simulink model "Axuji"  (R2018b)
settings: Solver=VariableStepAuto  StartTime=0.0  StopTime=1  RelTol=1e-3
libraries: fuzblock x6

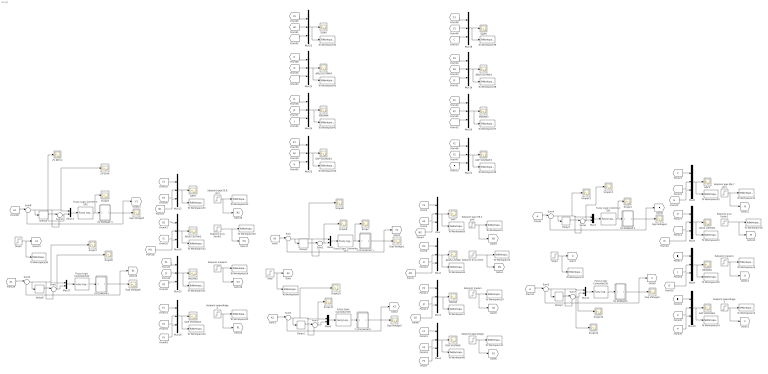
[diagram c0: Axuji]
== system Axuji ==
  2V EDMGAP 3 : Subsystem
  2V EDMGAP3 : Subsystem
  2V Error : Scope
  2V dError : Scope
  3.5V EDMGAP 1 : Subsystem
  3.5V EDMGAP2 : Subsystem
  5V EDMGAP 2 : Subsystem
  5V EDMGAP1 : Subsystem
  ARUS LISTRIK{,1..4} (5 alike) : Scope
  Delay{1..6} (6 alike) : Delay  DelayLength=1
  From11 : From
  From8 : From
  Fuzzy Logic Controller 3X1 : fuzblock/Fuzzy Logic  Controller  FIS=FixFUZZYSUGENO3X3  OutputSampleNumber=101  DataType=double  FuzzifiedInputs=off  RuleFiringStrengths=off  RuleOutputs=off  AggregatedOutputs=off  SimulateUsing=Interpreted execution  OutOfRangeInputValueMessage=warning  NoRuleFiredMessage=warning  EmptyOutputFuzzySetMessage=warning
  Fuzzy Logic Controller 3X2 : fuzblock/Fuzzy Logic  Controller  FIS=FixFUZZYSUGENO3X3  OutputSampleNumber=101  DataType=double  FuzzifiedInputs=off  RuleFiringStrengths=off  RuleOutputs=off  AggregatedOutputs=off  SimulateUsing=Interpreted execution  OutOfRangeInputValueMessage=warning  NoRuleFiredMessage=warning  EmptyOutputFuzzySetMessage=warning
  Fuzzy Logic Controller 3X3 : fuzblock/Fuzzy Logic  Controller  FIS=FixFUZZYSUGENO3X3  OutputSampleNumber=101  DataType=double  FuzzifiedInputs=off  RuleFiringStrengths=off  RuleOutputs=off  AggregatedOutputs=off  SimulateUsing=Interpreted execution  OutOfRangeInputValueMessage=warning  NoRuleFiredMessage=warning  EmptyOutputFuzzySetMessage=warning
  Fuzzy Logic Controller5X1 : fuzblock/Fuzzy Logic  Controller  FIS=FixFUZZYSUGENO5X5  OutputSampleNumber=101  DataType=double  FuzzifiedInputs=off  RuleFiringStrengths=off  RuleOutputs=off  AggregatedOutputs=off  SimulateUsing=Interpreted execution  OutOfRangeInputValueMessage=warning  NoRuleFiredMessage=warning  EmptyOutputFuzzySetMessage=warning
  Fuzzy Logic Controller5X2 : fuzblock/Fuzzy Logic  Controller  FIS=FixFUZZYSUGENO5X5  OutputSampleNumber=101  DataType=double  FuzzifiedInputs=off  RuleFiringStrengths=off  RuleOutputs=off  AggregatedOutputs=off  SimulateUsing=Interpreted execution  OutOfRangeInputValueMessage=warning  NoRuleFiredMessage=warning  EmptyOutputFuzzySetMessage=warning
  Fuzzy Logic Controller5X5 : fuzblock/Fuzzy Logic  Controller  FIS=FixFUZZYSUGENO5X5  OutputSampleNumber=101  DataType=double  FuzzifiedInputs=off  RuleFiringStrengths=off  RuleOutputs=off  AggregatedOutputs=off  SimulateUsing=Interpreted execution  OutOfRangeInputValueMessage=warning  NoRuleFiredMessage=warning  EmptyOutputFuzzySetMessage=warning
  GAP{,1..4} (5 alike) : Scope
  GAP VOLTAGE{,1..4} (5 alike) : Scope
  Gap Voltage{1..6} (6 alike) : Scope
  Goto7 : Goto
  MEDAN{,1..4} (5 alike) : Scope
  Mux{,2..4,6,8..10,12,14..16,18..25} (20 alike) : Mux  Inputs=3
  Mux{1,5,7,11,13,17} (6 alike) : Mux  Inputs=2
  Scope{,1..2,6..15} (13 alike) : Scope
  Setpoint arus listrik : Step  Time=0  After=0.00246  SampleTime=0
  Setpoint arus listrik1 : Step  Time=0  After=0.00246  SampleTime=0
  Setpoint arus listrik2 : Step  Time=0  After=0.00246  SampleTime=0
  Setpoint gap (59,3 µm) : Step  Time=0  After=59.3  SampleTime=0
  Setpoint gap (84,7 µm) : Step  Time=0  After=84.7  SampleTime=0
  Setpoint gap(33,8 µm) : Step  Time=0  After=33.8  SampleTime=0
  Setpoint gapvoltage : Step  Time=0  After=2  SampleTime=0
  Setpoint gapvoltage1 : Step  Time=0  After=2  SampleTime=0
  Setpoint gapvoltage2 : Step  Time=0  After=2  SampleTime=0
  Setpoint medan : Step  Time=0  After=59000  SampleTime=0
  Setpoint medan1 : Step  Time=0  After=59000  SampleTime=0
  Setpoint medan2 : Step  Time=0  After=59000  SampleTime=0
  Step : Step  Time=0  After=3.5  SampleTime=0
  Step1 : Step  Time=0  After=5  SampleTime=0
  Step2 : Step  Time=0  After=2  SampleTime=0
  Sum{,1..11} (12 alike) : Sum  Inputs=|-+
  To Workspace1 : ToWorkspace  VariableName=setpointgap  SaveFormat=Timeseries  SampleTime=-1
  To Workspace10 : ToWorkspace  VariableName=setpointmedan  SaveFormat=Timeseries  SampleTime=-1
  To Workspace11 : ToWorkspace  VariableName=setpointgvoltage  SaveFormat=Timeseries  SampleTime=-1
  To Workspace12 : ToWorkspace  VariableName=setpointgap1  SaveFormat=Timeseries  SampleTime=-1
  To Workspace13 : ToWorkspace  VariableName=setpointmedan1  SaveFormat=Timeseries  SampleTime=-1
  To Workspace14 : ToWorkspace  VariableName=setpointgvoltage1  SaveFormat=Timeseries  SampleTime=-1
  To Workspace17 : ToWorkspace  VariableName=setpoint1  SaveFormat=Timeseries  SampleTime=-1
  To Workspace18 : ToWorkspace  VariableName=setpointaruslistrik1  SaveFormat=Timeseries  SampleTime=-1
  To Workspace19 : ToWorkspace  VariableName=gapvoltage10  SaveFormat=Timeseries  SampleTime=-1
  To Workspace20 : ToWorkspace  VariableName=medan10  SaveFormat=Timeseries  SampleTime=-1
  To Workspace21 : ToWorkspace  VariableName=aruslistrik10  SaveFormat=Timeseries  SampleTime=-1
  To Workspace22 : ToWorkspace  VariableName=gap10  SaveFormat=Timeseries  SampleTime=-1
  To Workspace23 : ToWorkspace  VariableName=setpointgap2  SaveFormat=Timeseries  SampleTime=-1
  To Workspace24 : ToWorkspace  VariableName=setpointmedan2  SaveFormat=Timeseries  SampleTime=-1
  To Workspace25 : ToWorkspace  VariableName=setpointgvoltage2  SaveFormat=Timeseries  SampleTime=-1
  To Workspace28 : ToWorkspace  VariableName=setpoint2  SaveFormat=Timeseries  SampleTime=-1
  To Workspace29 : ToWorkspace  VariableName=setpointaruslistrik2  SaveFormat=Timeseries  SampleTime=-1
  To Workspace30 : ToWorkspace  VariableName=gapvoltage8  SaveFormat=Timeseries  SampleTime=-1
  To Workspace31 : ToWorkspace  VariableName=medan8  SaveFormat=Timeseries  SampleTime=-1
  To Workspace32 : ToWorkspace  VariableName=aruslistrik8  SaveFormat=Timeseries  SampleTime=-1
  To Workspace33 : ToWorkspace  VariableName=gap8  SaveFormat=Timeseries  SampleTime=-1
  To Workspace36 : ToWorkspace  VariableName=gapvoltage6  SaveFormat=Timeseries  SampleTime=-1
  To Workspace37 : ToWorkspace  VariableName=medan6  SaveFormat=Timeseries  SampleTime=-1
  To Workspace38 : ToWorkspace  VariableName=aruslistrik6  SaveFormat=Timeseries  SampleTime=-1
  To Workspace39 : ToWorkspace  VariableName=gap6  SaveFormat=Timeseries  SampleTime=-1
  To Workspace4 : ToWorkspace  VariableName=setpoint  SaveFormat=Timeseries  SampleTime=-1
  To Workspace40 : ToWorkspace  VariableName=gapvoltage7  SaveFormat=Timeseries  SampleTime=-1
  To Workspace41 : ToWorkspace  VariableName=medan7  SaveFormat=Timeseries  SampleTime=-1
  To Workspace42 : ToWorkspace  VariableName=aruslistrik7  SaveFormat=Timeseries  SampleTime=-1
  To Workspace43 : ToWorkspace  VariableName=gap7  SaveFormat=Timeseries  SampleTime=-1
  To Workspace5 : ToWorkspace  VariableName=setpointaruslistrik  SaveFormat=Timeseries  SampleTime=-1
  To Workspace6 : ToWorkspace  VariableName=gapvoltage9  SaveFormat=Timeseries  SampleTime=-1
  To Workspace7 : ToWorkspace  VariableName=medan9  SaveFormat=Timeseries  SampleTime=-1
  To Workspace8 : ToWorkspace  VariableName=aruslistrik9  SaveFormat=Timeseries  SampleTime=-1
  To Workspace9 : ToWorkspace  VariableName=gap9  SaveFormat=Timeseries  SampleTime=-1
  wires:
  [N2] -> Mux/3
  Setpoint gapvoltage/1 -> [P2], To Workspace11/1
  [I2] -> Mux2/2
  [D2] -> Mux2/1
  Sum2/1 -> Scope9/1, Mux1/2
  Mux5/1 -> Fuzzy Logic Controller5X5/1
  [O2] -> Mux3/3
  Delay2/1 -> Sum3/1
  [H2] -> Mux/2
  Mux/1 -> To Workspace9/1, GAP/1
  Setpoint arus listrik/1 -> [M2], To Workspace5/1
  Setpoint medan/1 -> [O2], To Workspace10/1
  Sum/1 -> Delay1/1, Scope8/1, Sum2/2, Mux1/1
  [M2] -> Mux2/3
  Delay1/1 -> Sum2/1
  [K2] -> Mux4/2
  [J2] -> Mux3/2
  [F2] -> Mux4/1
  Mux1/1 -> Fuzzy Logic Controller 3X3/1
  Fuzzy Logic Controller 3X3/1 -> Scope/1, 3.5V EDMGAP 1/1(In1)
  Mux4/1 -> To Workspace6/1, GAP VOLTAGE/1
  [A2] -> Sum1/1
  Setpoint gap (59,3 µm)/1 -> [N2], To Workspace1/1
  Mux3/1 -> To Workspace7/1, MEDAN/1
  [E2] -> Mux3/1
  Sum1/1 -> Delay2/1, Scope10/1, Sum3/2, Mux5/1
  Step/1 -> To Workspace4/1, [A2]
  Mux2/1 -> To Workspace8/1, ARUS LISTRIK/1
  Sum3/1 -> Scope11/1, Mux5/2
  [C2] -> Mux/1
  [A2] -> Sum/1
  [P2] -> Mux4/3
  3.5V EDMGAP2/1(Out1) -> [K2], Gap Voltage2/1, Sum1/2
  3.5V EDMGAP 1/1(Out1) -> Sum/2, Gap Voltage1/1, [F2]
  Fuzzy Logic Controller5X5/1 -> 3.5V EDMGAP2/1(In1)
  5V EDMGAP1/1(Out1) -> [K], Gap Voltage4/1, Sum5/2
  [J] -> Mux9/2
  Setpoint gapvoltage1/1 -> [P], To Workspace14/1
  Fuzzy Logic Controller5X1/1 -> 5V EDMGAP1/1(In1)
  [H] -> Mux6/2
  [N] -> Mux6/3
  [C] -> Mux6/1
  Mux6/1 -> To Workspace22/1, GAP1/1
  [F] -> Mux10/1
  Sum7/1 -> Scope15/1, Mux11/2
  Mux9/1 -> To Workspace20/1, MEDAN1/1
  Mux8/1 -> To Workspace21/1, ARUS LISTRIK1/1
  Sum5/1 -> Delay4/1, Sum7/2, Scope14/1, Mux11/1
  [P] -> Mux10/3
  Mux7/1 -> Fuzzy Logic Controller 3X1/1
  [O] -> Mux9/3
  Step1/1 -> To Workspace17/1, Goto7/1
  From11/1 -> Sum5/1
  [I] -> Mux8/2
  Mux10/1 -> To Workspace19/1, GAP VOLTAGE1/1
  Fuzzy Logic Controller 3X1/1 -> Scope1/1, 5V EDMGAP 2/1(In1)
  [K] -> Mux10/2
  [M] -> Mux8/3
  Setpoint arus listrik1/1 -> [M], To Workspace18/1
  Delay3/1 -> Sum6/1
  Setpoint gap (84,7 µm)/1 -> [N], To Workspace12/1
  5V EDMGAP 2/1(Out1) -> Sum4/2, Gap Voltage3/1, [F]
  [E] -> Mux9/1
  Delay4/1 -> Sum7/1
  Sum6/1 -> Scope13/1, Mux7/2
  Setpoint medan1/1 -> [O], To Workspace13/1
  From8/1 -> Sum4/1
  [D] -> Mux8/1
  Sum4/1 -> Delay3/1, Scope12/1, Sum6/2, Mux7/1
  Mux11/1 -> Fuzzy Logic Controller5X1/1
  2V EDMGAP3/1(Out1) -> [K1], Gap Voltage6/1, Sum9/2
  [J1] -> Mux15/2
  Setpoint gapvoltage2/1 -> [P1], To Workspace25/1
  Fuzzy Logic Controller5X2/1 -> 2V EDMGAP3/1(In1)
  [H1] -> Mux12/2
  [N1] -> Mux12/3
  [C1] -> Mux12/1
  Mux12/1 -> To Workspace33/1, GAP2/1
  [F1] -> Mux16/1
  Sum11/1 -> Scope6/1, Mux17/2
  Mux15/1 -> To Workspace31/1, MEDAN2/1
  Mux14/1 -> To Workspace32/1, ARUS LISTRIK2/1
  Sum9/1 -> Delay6/1, Sum11/2, Scope7/1, Mux17/1
  [P1] -> Mux16/3
  Mux13/1 -> Fuzzy Logic Controller 3X2/1
  [O1] -> Mux15/3
  Step2/1 -> To Workspace28/1, [A1]
  [A1] -> Sum9/1
  [I1] -> Mux14/2
  Mux16/1 -> To Workspace30/1, GAP VOLTAGE2/1
  Fuzzy Logic Controller 3X2/1 -> Scope2/1, 2V EDMGAP 3/1(In1)
  [K1] -> Mux16/2
  [M1] -> Mux14/3
  Setpoint arus listrik2/1 -> [M1], To Workspace29/1
  Delay5/1 -> Sum10/1
  Setpoint gap(33,8 µm)/1 -> [N1], To Workspace23/1
  2V EDMGAP 3/1(Out1) -> Sum8/2, Gap Voltage5/1, [F1]
  [E1] -> Mux15/1
  Delay6/1 -> Sum11/1
  Sum10/1 -> 2V dError/1, Mux13/2
  Setpoint medan2/1 -> [O1], To Workspace24/1
  [A1] -> Sum8/1
  [D1] -> Mux14/1
  Sum8/1 -> Delay5/1, Sum10/2, 2V Error/1, Mux13/1
  Mux17/1 -> Fuzzy Logic Controller5X2/1
  [D2] -> Mux19/2
  [F1] -> Mux21/1
  Mux21/1 -> To Workspace36/1, GAP VOLTAGE3/1
  Mux20/1 -> To Workspace37/1, MEDAN3/1
  Mux18/1 -> To Workspace39/1, GAP3/1
  [F] -> Mux21/3
  [C2] -> Mux18/2
  [E2] -> Mux20/2
  [F2] -> Mux21/2
  [E1] -> Mux20/1
  [D] -> Mux19/3
  [C] -> Mux18/3
  Mux19/1 -> To Workspace38/1, ARUS LISTRIK3/1
  [E] -> Mux20/3
  [C1] -> Mux18/1
  [D1] -> Mux19/1
  [I2] -> Mux23/2
  [K1] -> Mux25/1
  Mux25/1 -> To Workspace40/1, GAP VOLTAGE4/1
  Mux24/1 -> To Workspace41/1, MEDAN4/1
  Mux22/1 -> To Workspace43/1, GAP4/1
  [K] -> Mux25/3
  [H2] -> Mux22/2
  [J2] -> Mux24/2
  [K2] -> Mux25/2
  [J1] -> Mux24/1
  [I] -> Mux23/3
  [H] -> Mux22/3
  Mux23/1 -> To Workspace42/1, ARUS LISTRIK4/1
  [J] -> Mux24/3
  [H1] -> Mux22/1
  [I1] -> Mux23/1

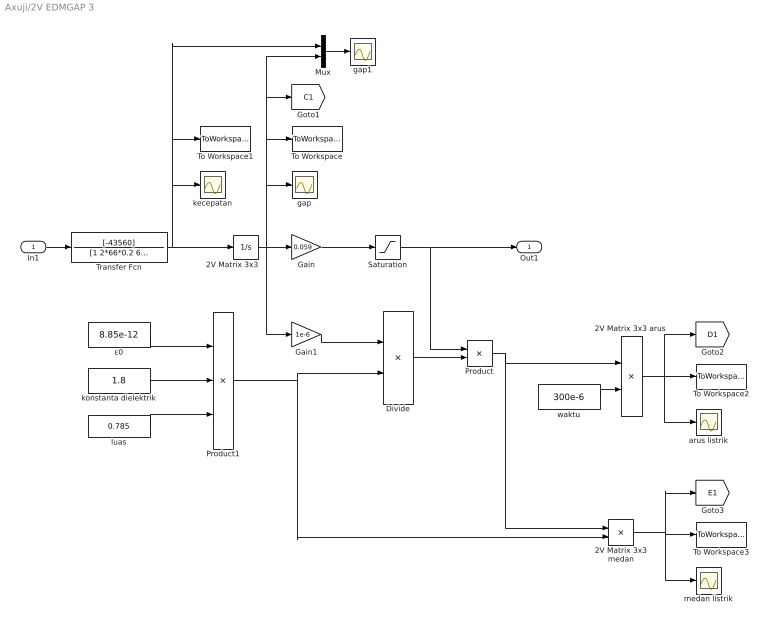
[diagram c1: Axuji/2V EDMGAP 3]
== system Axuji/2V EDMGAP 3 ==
  In1 : Inport
  2V Matrix 3x3 : Integrator  InitialCondition=225
  "2V Matrix 3x3 arus " : Product  Inputs=*/
  2V Matrix 3x3 medan : Product  Inputs=*/
  Divide : Product  Inputs=/*
  Gain : Gain  Gain=0.059
  Gain1 : Gain  Gain=1e-6
  Mux : Mux  Inputs=2
  Product : Product
  Product1 : Product  Inputs=3
  Saturation : Saturate  UpperLimit=10  LowerLimit=0
  To Workspace : ToWorkspace  VariableName=gap  SaveFormat=Timeseries  SampleTime=-1
  To Workspace1 : ToWorkspace  VariableName=kecepatan  SaveFormat=Timeseries  SampleTime=-1
  To Workspace2 : ToWorkspace  VariableName=aruslistrik  SaveFormat=Timeseries  SampleTime=-1
  To Workspace3 : ToWorkspace  VariableName=medan  SaveFormat=Timeseries  SampleTime=-1
  Transfer Fcn : TransferFcn  Numerator=[-43560]  Denominator=[1 2*66*0.2 66^2]
  arus listrik : Scope
  gap : Scope
  gap1 : Scope
  kecepatan : Scope
  konstanta dielektrik : Constant  Value=1.8
  luas : Constant  Value=0.785
  medan listrik : Scope
  waktu : Constant  Value=300e-6
  ε0 : Constant  Value=8.85e-12
  Out1 : Outport
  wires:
  2V Matrix 3x3/1 -> Gain1/1, Mux/2, [C1], To Workspace/1, gap/1, Gain/1
  In1/1 -> Transfer Fcn/1
  Gain1/1 -> Divide/1
  Product1/1 -> 2V Matrix 3x3 medan/2, Divide/2
  ε0/1 -> Product1/1
  konstanta dielektrik/1 -> Product1/2
  luas/1 -> Product1/3
  Divide/1 -> Product/2
  Product/1 -> 2V Matrix 3x3 medan/1, "2V Matrix 3x3 arus "/1
  waktu/1 -> "2V Matrix 3x3 arus "/2
  "2V Matrix 3x3 arus "/1 -> arus listrik/1, [D1], To Workspace2/1
  2V Matrix 3x3 medan/1 -> medan listrik/1, [E1], To Workspace3/1
  Mux/1 -> gap1/1
  Transfer Fcn/1 -> Mux/1, To Workspace1/1, kecepatan/1, 2V Matrix 3x3/1
  Saturation/1 -> Product/1, Out1/1
  Gain/1 -> Saturation/1

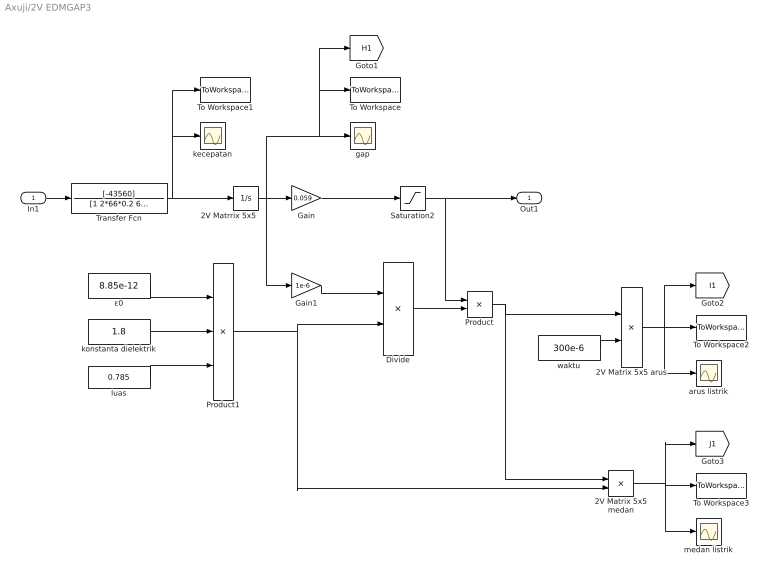
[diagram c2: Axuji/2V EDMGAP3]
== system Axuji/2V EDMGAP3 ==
  In1 : Inport
  2V Matrix 5x5 arus : Product  Inputs=*/
  2V Matrix 5x5 medan : Product  Inputs=*/
  "2V Matrrix 5x5 " : Integrator  InitialCondition=225
  Divide : Product  Inputs=/*
  Gain : Gain  Gain=0.059
  Gain1 : Gain  Gain=1e-6
  Product : Product
  Product1 : Product  Inputs=3
  Saturation2 : Saturate  UpperLimit=10  LowerLimit=0
  To Workspace : ToWorkspace  VariableName=gap1  SaveFormat=Timeseries  SampleTime=-1
  To Workspace1 : ToWorkspace  VariableName=kecepatan1  SaveFormat=Timeseries  SampleTime=-1
  To Workspace2 : ToWorkspace  VariableName=aruslistrik1  SaveFormat=Timeseries  SampleTime=-1
  To Workspace3 : ToWorkspace  VariableName=medan1  SaveFormat=Timeseries  SampleTime=-1
  Transfer Fcn : TransferFcn  Numerator=[-43560]  Denominator=[1 2*66*0.2 66^2]
  arus listrik : Scope
  gap : Scope
  kecepatan : Scope
  konstanta dielektrik : Constant  Value=1.8
  luas : Constant  Value=0.785
  medan listrik : Scope
  waktu : Constant  Value=300e-6
  ε0 : Constant  Value=8.85e-12
  Out1 : Outport
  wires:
  In1/1 -> Transfer Fcn/1
  Transfer Fcn/1 -> To Workspace1/1, kecepatan/1, "2V Matrrix 5x5 "/1
  Gain1/1 -> Divide/1
  Product1/1 -> 2V Matrix 5x5 medan/2, Divide/2
  ε0/1 -> Product1/1
  konstanta dielektrik/1 -> Product1/2
  luas/1 -> Product1/3
  Divide/1 -> Product/2
  Product/1 -> 2V Matrix 5x5 medan/1, 2V Matrix 5x5 arus/1
  waktu/1 -> 2V Matrix 5x5 arus/2
  2V Matrix 5x5 arus/1 -> arus listrik/1, [I1], To Workspace2/1
  2V Matrix 5x5 medan/1 -> medan listrik/1, [J1], To Workspace3/1
  "2V Matrrix 5x5 "/1 -> [H1], To Workspace/1, gap/1, Gain1/1, Gain/1
  Saturation2/1 -> Product/1, Out1/1
  Gain/1 -> Saturation2/1

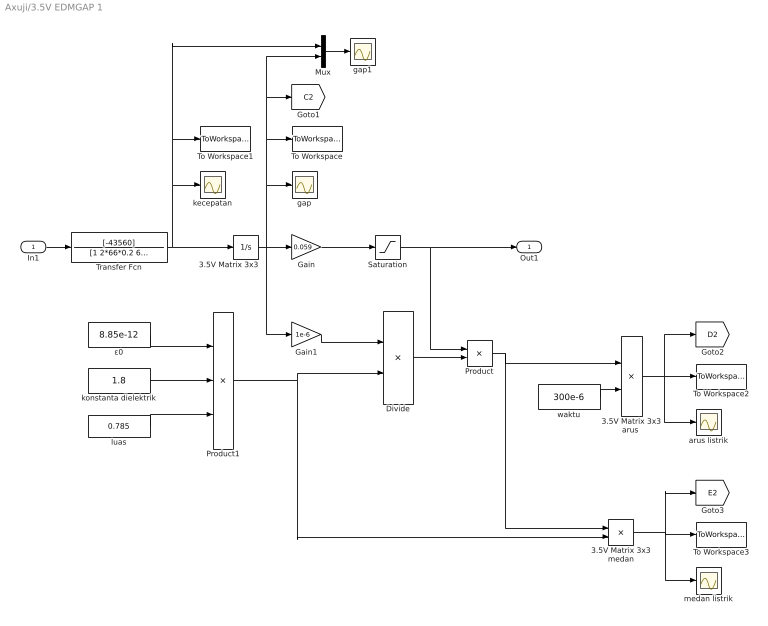
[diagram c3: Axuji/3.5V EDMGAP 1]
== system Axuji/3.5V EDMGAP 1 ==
  In1 : Inport
  3.5V Matrix 3x3 : Integrator  InitialCondition=225
  "3.5V Matrix 3x3 arus " : Product  Inputs=*/
  3.5V Matrix 3x3 medan : Product  Inputs=*/
  Divide : Product  Inputs=/*
  Gain : Gain  Gain=0.059
  Gain1 : Gain  Gain=1e-6
  Mux : Mux  Inputs=2
  Product : Product
  Product1 : Product  Inputs=3
  Saturation : Saturate  UpperLimit=10  LowerLimit=0
  To Workspace : ToWorkspace  VariableName=gap2  SaveFormat=Timeseries  SampleTime=-1
  To Workspace1 : ToWorkspace  VariableName=kecepatan2  SaveFormat=Timeseries  SampleTime=-1
  To Workspace2 : ToWorkspace  VariableName=aruslistrik2  SaveFormat=Timeseries  SampleTime=-1
  To Workspace3 : ToWorkspace  VariableName=medan2  SaveFormat=Timeseries  SampleTime=-1
  Transfer Fcn : TransferFcn  Numerator=[-43560]  Denominator=[1 2*66*0.2 66^2]
  arus listrik : Scope
  gap : Scope
  gap1 : Scope
  kecepatan : Scope
  konstanta dielektrik : Constant  Value=1.8
  luas : Constant  Value=0.785
  medan listrik : Scope
  waktu : Constant  Value=300e-6
  ε0 : Constant  Value=8.85e-12
  Out1 : Outport
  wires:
  3.5V Matrix 3x3/1 -> Gain1/1, Mux/2, [C2], To Workspace/1, gap/1, Gain/1
  In1/1 -> Transfer Fcn/1
  Gain1/1 -> Divide/1
  Product1/1 -> 3.5V Matrix 3x3 medan/2, Divide/2
  ε0/1 -> Product1/1
  konstanta dielektrik/1 -> Product1/2
  luas/1 -> Product1/3
  Divide/1 -> Product/2
  Product/1 -> 3.5V Matrix 3x3 medan/1, "3.5V Matrix 3x3 arus "/1
  waktu/1 -> "3.5V Matrix 3x3 arus "/2
  "3.5V Matrix 3x3 arus "/1 -> arus listrik/1, [D2], To Workspace2/1
  3.5V Matrix 3x3 medan/1 -> medan listrik/1, [E2], To Workspace3/1
  Mux/1 -> gap1/1
  Transfer Fcn/1 -> Mux/1, To Workspace1/1, kecepatan/1, 3.5V Matrix 3x3/1
  Saturation/1 -> Product/1, Out1/1
  Gain/1 -> Saturation/1

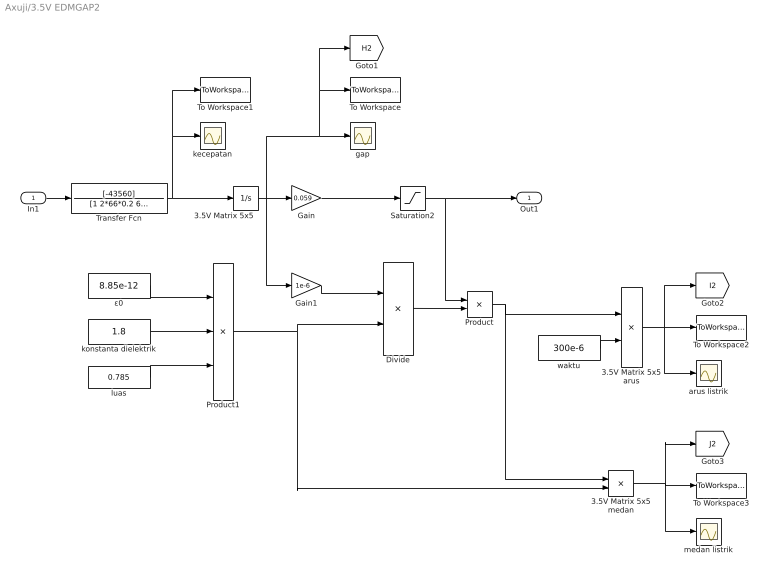
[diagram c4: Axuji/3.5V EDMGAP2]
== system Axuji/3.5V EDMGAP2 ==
  In1 : Inport
  "3.5V Matrix 5x5  " : Integrator  InitialCondition=225
  3.5V Matrix 5x5 arus : Product  Inputs=*/
  3.5V Matrix 5x5 medan : Product  Inputs=*/
  Divide : Product  Inputs=/*
  Gain : Gain  Gain=0.059
  Gain1 : Gain  Gain=1e-6
  Product : Product
  Product1 : Product  Inputs=3
  Saturation2 : Saturate  UpperLimit=10  LowerLimit=0
  To Workspace : ToWorkspace  VariableName=gap3  SaveFormat=Timeseries  SampleTime=-1
  To Workspace1 : ToWorkspace  VariableName=kecepatan3  SaveFormat=Timeseries  SampleTime=-1
  To Workspace2 : ToWorkspace  VariableName=aruslistrik3  SaveFormat=Timeseries  SampleTime=-1
  To Workspace3 : ToWorkspace  VariableName=medan3  SaveFormat=Timeseries  SampleTime=-1
  Transfer Fcn : TransferFcn  Numerator=[-43560]  Denominator=[1 2*66*0.2 66^2]
  arus listrik : Scope
  gap : Scope
  kecepatan : Scope
  konstanta dielektrik : Constant  Value=1.8
  luas : Constant  Value=0.785
  medan listrik : Scope
  waktu : Constant  Value=300e-6
  ε0 : Constant  Value=8.85e-12
  Out1 : Outport
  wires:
  In1/1 -> Transfer Fcn/1
  Transfer Fcn/1 -> To Workspace1/1, kecepatan/1, "3.5V Matrix 5x5  "/1
  Gain1/1 -> Divide/1
  Product1/1 -> 3.5V Matrix 5x5 medan/2, Divide/2
  ε0/1 -> Product1/1
  konstanta dielektrik/1 -> Product1/2
  luas/1 -> Product1/3
  Divide/1 -> Product/2
  Product/1 -> 3.5V Matrix 5x5 medan/1, 3.5V Matrix 5x5 arus/1
  waktu/1 -> 3.5V Matrix 5x5 arus/2
  3.5V Matrix 5x5 arus/1 -> arus listrik/1, [I2], To Workspace2/1
  3.5V Matrix 5x5 medan/1 -> medan listrik/1, [J2], To Workspace3/1
  "3.5V Matrix 5x5  "/1 -> [H2], To Workspace/1, gap/1, Gain1/1, Gain/1
  Saturation2/1 -> Product/1, Out1/1
  Gain/1 -> Saturation2/1

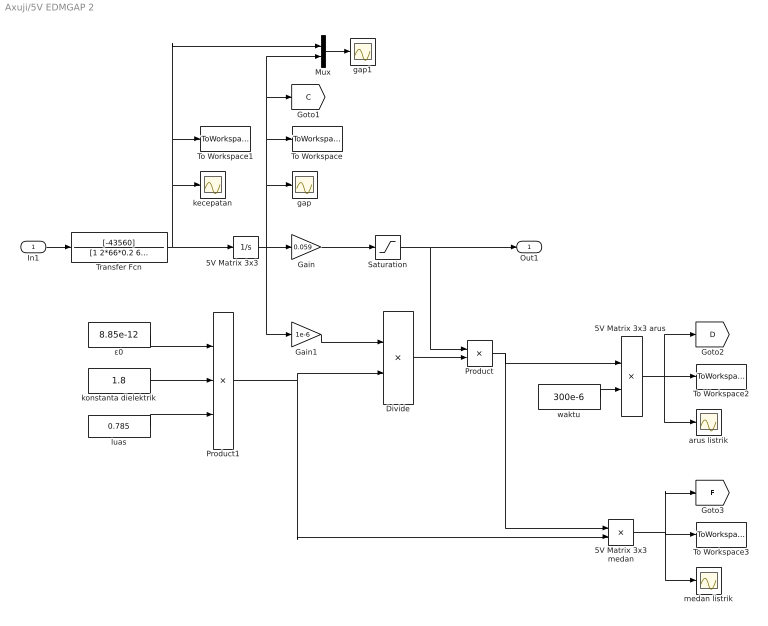
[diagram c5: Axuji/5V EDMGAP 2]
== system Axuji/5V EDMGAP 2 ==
  In1 : Inport
  5V Matrix 3x3 : Integrator  InitialCondition=225
  "5V Matrix 3x3 arus " : Product  Inputs=*/
  5V Matrix 3x3 medan : Product  Inputs=*/
  Divide : Product  Inputs=/*
  Gain : Gain  Gain=0.059
  Gain1 : Gain  Gain=1e-6
  Mux : Mux  Inputs=2
  Product : Product
  Product1 : Product  Inputs=3
  Saturation : Saturate  UpperLimit=10  LowerLimit=0
  To Workspace : ToWorkspace  VariableName=gap4  SaveFormat=Timeseries  SampleTime=-1
  To Workspace1 : ToWorkspace  VariableName=kecepatan4  SaveFormat=Timeseries  SampleTime=-1
  To Workspace2 : ToWorkspace  VariableName=aruslistrik4  SaveFormat=Timeseries  SampleTime=-1
  To Workspace3 : ToWorkspace  VariableName=medan4  SaveFormat=Timeseries  SampleTime=-1
  Transfer Fcn : TransferFcn  Numerator=[-43560]  Denominator=[1 2*66*0.2 66^2]
  arus listrik : Scope
  gap : Scope
  gap1 : Scope
  kecepatan : Scope
  konstanta dielektrik : Constant  Value=1.8
  luas : Constant  Value=0.785
  medan listrik : Scope
  waktu : Constant  Value=300e-6
  ε0 : Constant  Value=8.85e-12
  Out1 : Outport
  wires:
  5V Matrix 3x3/1 -> Gain1/1, Mux/2, [C], To Workspace/1, gap/1, Gain/1
  In1/1 -> Transfer Fcn/1
  Gain1/1 -> Divide/1
  Product1/1 -> 5V Matrix 3x3 medan/2, Divide/2
  ε0/1 -> Product1/1
  konstanta dielektrik/1 -> Product1/2
  luas/1 -> Product1/3
  Divide/1 -> Product/2
  Product/1 -> 5V Matrix 3x3 medan/1, "5V Matrix 3x3 arus "/1
  waktu/1 -> "5V Matrix 3x3 arus "/2
  "5V Matrix 3x3 arus "/1 -> arus listrik/1, [D], To Workspace2/1
  5V Matrix 3x3 medan/1 -> medan listrik/1, [E], To Workspace3/1
  Mux/1 -> gap1/1
  Transfer Fcn/1 -> Mux/1, To Workspace1/1, kecepatan/1, 5V Matrix 3x3/1
  Saturation/1 -> Product/1, Out1/1
  Gain/1 -> Saturation/1

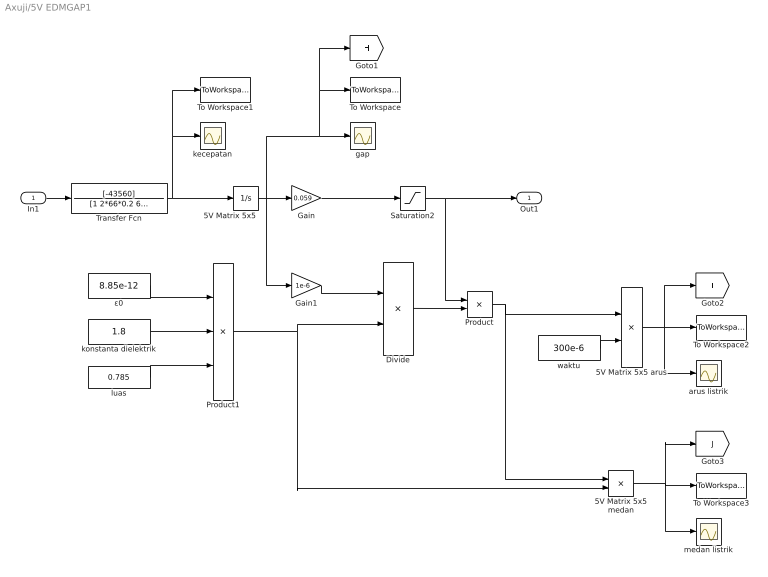
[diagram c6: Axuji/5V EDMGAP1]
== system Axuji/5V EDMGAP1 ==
  In1 : Inport
  "5V Matrix 5x5 " : Integrator  InitialCondition=225
  5V Matrix 5x5 arus : Product  Inputs=*/
  5V Matrix 5x5 medan : Product  Inputs=*/
  Divide : Product  Inputs=/*
  Gain : Gain  Gain=0.059
  Gain1 : Gain  Gain=1e-6
  Product : Product
  Product1 : Product  Inputs=3
  Saturation2 : Saturate  UpperLimit=10  LowerLimit=0
  To Workspace : ToWorkspace  VariableName=gap5  SaveFormat=Timeseries  SampleTime=-1
  To Workspace1 : ToWorkspace  VariableName=kecepatan5  SaveFormat=Timeseries  SampleTime=-1
  To Workspace2 : ToWorkspace  VariableName=aruslistrik5  SaveFormat=Timeseries  SampleTime=-1
  To Workspace3 : ToWorkspace  VariableName=medan5  SaveFormat=Timeseries  SampleTime=-1
  Transfer Fcn : TransferFcn  Numerator=[-43560]  Denominator=[1 2*66*0.2 66^2]
  arus listrik : Scope
  gap : Scope
  kecepatan : Scope
  konstanta dielektrik : Constant  Value=1.8
  luas : Constant  Value=0.785
  medan listrik : Scope
  waktu : Constant  Value=300e-6
  ε0 : Constant  Value=8.85e-12
  Out1 : Outport
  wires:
  In1/1 -> Transfer Fcn/1
  Transfer Fcn/1 -> To Workspace1/1, kecepatan/1, "5V Matrix 5x5 "/1
  Gain1/1 -> Divide/1
  Product1/1 -> 5V Matrix 5x5 medan/2, Divide/2
  ε0/1 -> Product1/1
  konstanta dielektrik/1 -> Product1/2
  luas/1 -> Product1/3
  Divide/1 -> Product/2
  Product/1 -> 5V Matrix 5x5 medan/1, 5V Matrix 5x5 arus/1
  waktu/1 -> 5V Matrix 5x5 arus/2
  5V Matrix 5x5 arus/1 -> arus listrik/1, [I], To Workspace2/1
  5V Matrix 5x5 medan/1 -> medan listrik/1, [J], To Workspace3/1
  "5V Matrix 5x5 "/1 -> [H], To Workspace/1, gap/1, Gain1/1, Gain/1
  Saturation2/1 -> Product/1, Out1/1
  Gain/1 -> Saturation2/1
